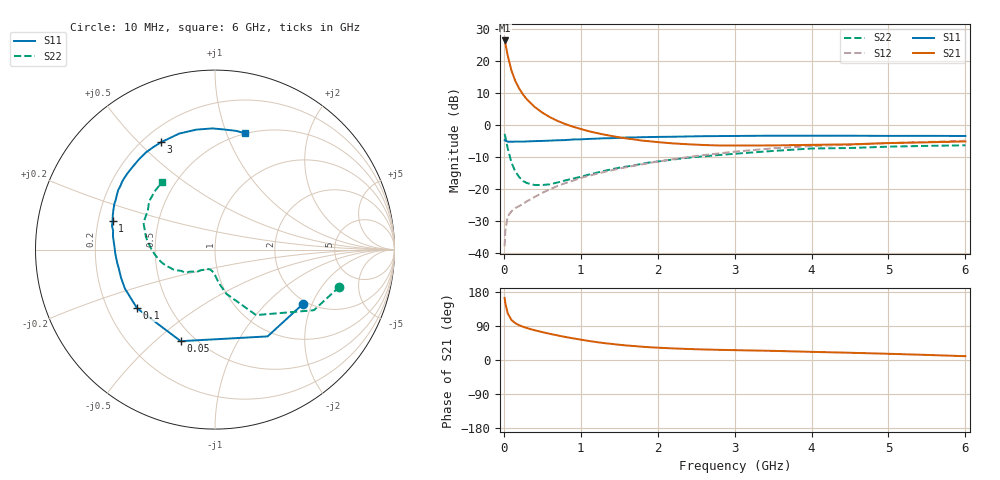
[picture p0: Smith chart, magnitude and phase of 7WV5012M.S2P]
! Infineon Technologies  Discrete & RF Semiconductors
! BFS17W
! Si NPN RF Bipolar Junction Transistor in SOT323
! VCE = 0.5 V  IC = 12 mA
! Common Emitter S-Parameters:  August  1999
# GHz  S  MA  R  50
!  f  S11  S21  S12  S22
! GHz  MAG  ANG  MAG  ANG  MAG  ANG  MAG  ANG
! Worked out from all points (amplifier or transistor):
!   36 points, 10 MHz to 6 GHz, reference 50 ohm
!   highest |S21| = 26.4 dB at 10 MHz (marker M1)
!   |S21| within 3 dB of that: start of sweep to 36.57 MHz
!   unconditionally stable (mu >= 1): 90.26 MHz to end of sweep
!   at 250 MHz: K = 2.03, MAG = 11.3 dB, |S12| = -24.8 dB
!   at 1.4 GHz: K = 2.34, MAG = -1.1 dB, |S12| = -14.2 dB
!   at 6 GHz: K = 1.16, MAG = -2.5 dB, |S12| = -5.0 dB
!   S11 on the Smith chart (normalised r, x): 10 MHz: 1.91, -1.72; 50 MHz: 0.42, -0.61; 100 MHz: 0.33, -0.30; 1 GHz: 0.26, +0.13; 3 GHz: 0.27, +0.58; 6 GHz: 0.50, +1.16
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0.01  0.5765 -31.6  20.94 163.8  0.0126 74.7  0.7234 -16.6
0.02  0.5654 -58.8  18.82 149.6  0.0222 62.4  0.6464 -31.5
0.05  0.5447 -110.5  12.21 123.1  0.037 43.0  0.4307 -57.9
0.1  0.5434 -143.0  7.016 105.3  0.0443 35.8  0.2542 -75.6
0.15  0.5468 -156.5  4.821 97.0  0.0497 36.9  0.1855 -83.8
0.2  0.5465 -163.5  3.689 91.7  0.0536 40.5  0.1518 -88.2
0.25  0.546 -168.6  2.971 87.7  0.0578 42.9  0.1318 -92.6
0.3  0.5497 -172.1  2.504 84.3  0.0636 46.0  0.1226 -96.4
0.4  0.5558 -177.5  1.908 78.5  0.0742 50.3  0.1143 -103.3
0.5  0.5601 178.6  1.553 73.6  0.0862 53.7  0.1144 -107.3
0.6  0.566 175.5  1.316 69.0  0.098 55.5  0.1172 -112.1
0.8  0.5774 169.5  1.027 60.7  0.1224 57.6  0.135 -122.3
1  0.5926 164.3  0.861 53.8  0.1472 58.4  0.1533 -127.6
1.1  0.6017 161.1  0.797 50.4  0.1587 58.3  0.1661 -132.3
1.3  0.6156 155.7  0.705 44.7  0.1826 57.8  0.1893 -139.3
1.6  0.6333 148.4  0.611 38.2  0.2178 56.5  0.2227 -147.8
2.2  0.6511 134.3  0.512 30.6  0.2896 52.4  0.2866 -161.7
3  0.6694 116.6  0.474 26.0  0.3804 44.2  0.3525 -179.7
3.5  0.6765 107.1  0.476 24.1  0.4292 38.3  0.3902 170.0
4.5  0.6754 91.1  0.495 19.1  0.4883 26.8  0.4335 149.6
5.5  0.672 79.9  0.532 13.4  0.5394 17.9  0.468 135.2
6  0.6692 75.5  0.55 10.0  0.5626 13.5  0.4783 128.0
